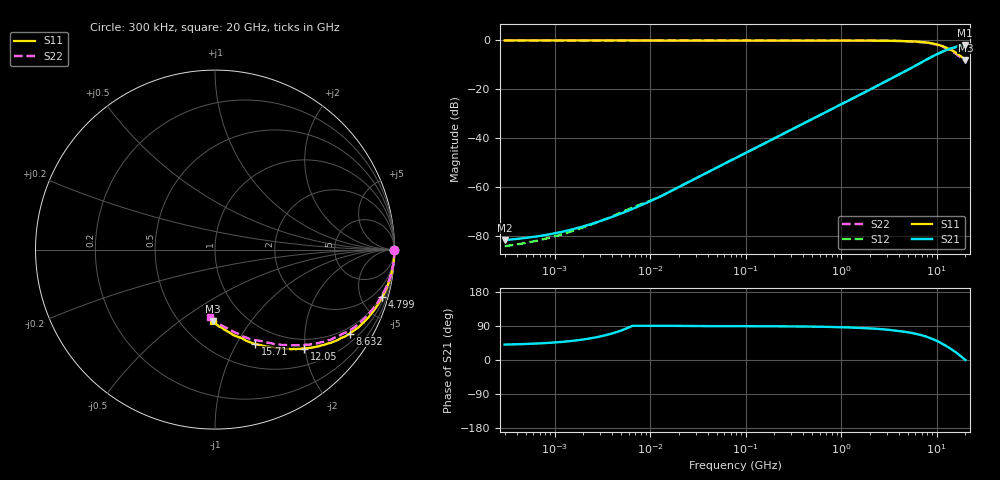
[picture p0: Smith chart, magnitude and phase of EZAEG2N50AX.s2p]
!*** S-Parameter ***
!Copyright (C)  Panasonic Industry
!ESD Suppressor
!Parts No.  EZAEG2N50AX
! Size : 1005mm
# hz S ma R 50
! 2 Port Network Data from SP1.SP block
! freq  magS11  angS11  magS21  angS21  magS12  angS12  magS22  angS22
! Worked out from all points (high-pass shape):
!   966 points, 300 kHz to 20 GHz, reference 50 ohm
!   highest |S21| = -1.85 dB at 19.77 GHz (marker M1); lowest = -81.7 dB at 300 kHz (marker M2)
!   |S21| within 3 dB of the highest: 11.05 GHz to end of sweep
!   lowest |S11| = -8.0 dB at 20 GHz (marker M3), VSWR 2.33, Z = 35.6 - j33.7 ohm
!   |S11| at or under -10 dB: nowhere
!   |S22| runs from -8.5 to 0.0 dB; largest |S21 - S12| = 0.022
!   S11 on the Smith chart (normalised r, x): 300 kHz: open; 4.799 GHz: 0.83, -7.09; 8.632 GHz: 0.77, -3.34; 12.05 GHz: 0.81, -1.98; 15.71 GHz: 0.77, -1.20; 20 GHz: 0.71, -0.67
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300000  0.9999 0.0  8.255e-05 40.7  6.196e-05 -10.3  1 0.0
687131.5  0.9999 0.0  9.961e-05 43.8  8.192e-05 -4.3  0.9999 0.0
1028017  0.9999 0.0  0.0001146 46.5  9.95e-05 1.0  0.9999 0.0
1913988  0.9998 0.0  0.0001537 53.5  0.0001452 14.6  0.9999 0.0
2964123  0.9998 0.0  0.0001999 61.8  0.0001994 30.9  0.9999 0.0
4697329  0.9999 -0.0  0.0002763 75.5  0.0002887 57.7  0.9999 -0.0
1.221117e7  0.9999 -0.0  0.0006149 90.3  0.0006178 91.0  1 -0.0
7.790674e7  0.9994 -0.2  0.003894 89.3  0.003897 89.2  1 -0.2
4.970419e8  0.9991 -1.5  0.02461 88.1  0.02462 88.0  0.9996 -1.4
1.433141e9  0.9967 -4.4  0.07073 85.2  0.07069 85.1  0.997 -4.3
2.219453e9  0.9931 -7.0  0.1097 82.7  0.1096 82.5  0.9927 -6.7
3.171107e9  0.9867 -10.1  0.1574 79.6  0.157 79.3  0.9847 -9.8
4.799215e9  0.9687 -15.9  0.2409 73.8  0.2402 73.4  0.9651 -15.3
6.624278e9  0.9382 -23.0  0.3395 66.6  0.337 66.4  0.93 -22.3
8.632022e9  0.8852 -31.9  0.4517 57.3  0.4453 57.6  0.8752 -31.0
1.049768e10  0.8114 -40.6  0.5457 47.9  0.5379 48.0  0.7965 -40.1
1.205257e10  0.7414 -48.0  0.6143 39.6  0.6021 39.9  0.7174 -47.8
1.399797e10  0.6493 -57.9  0.6822 29.8  0.6728 30.6  0.6208 -58.1
1.570557e10  0.5708 -66.9  0.7342 21.4  0.721 21.6  0.5421 -67.5
1.762148e10  0.4882 -77.7  0.7787 11.2  0.7624 11.9  0.4563 -79.1
1.977111e10  0.4084 -90.3  0.8085 0.8  0.7907 1.6  0.3832 -93.7
2e10  0.3986 -91.7  0.8072 -0.1  0.791 0.5  0.3765 -94.6
